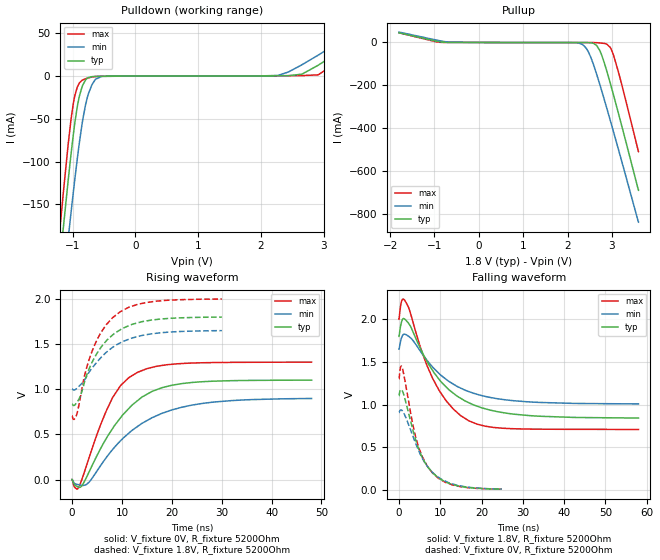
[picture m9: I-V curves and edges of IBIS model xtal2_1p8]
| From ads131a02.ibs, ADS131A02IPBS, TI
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|   xtal2_1p8 Model
[Model]   xtal2_1p8
Model_type   Output
Polarity   Inverting
Vmeas = 0.9
Vref = 0
Cref = 2pF
Rref = 5200
|   typ   min   max
|   (nom PVT)   (fast PVT)   (slow PVT)
C_comp   1.642e-12   1.633e-12   1.659e-12
| Where nom  PVT is Nominal Process, 1.8V, 27C
|   Fast PVT is Strong Process,  2V, -40C
|   Slow PVT is Weak Process,   1.65V, 125C
[Voltage Range]   1.8   1.65   2
|Junction Temperature
[Temperature Range]   27   125   -40
[Pullup Reference]   1.8   1.65   2
[Pulldown Reference]   0   0   0
[Power Clamp Reference]   1.8   1.65   2
[GND Clamp Reference]   0   0   0
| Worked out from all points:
|   slope of the pulldown table from 0 to 0.27 V, typ, clamps not added: 3.11 kohm
|   slope of the pullup table from 0 to 0.27 V, typ, clamps not added: 3.11 kohm
|   falling waveform, V_fixture 1.8V, R_fixture 5200Ohm: 20-80 % time 10.7ns typ, 11.1ns min, 8.07ns max; typ from 1.8 V to 0.842 V
|   rising waveform, V_fixture 0V, R_fixture 5200Ohm: 20-80 % time 8.7ns typ, 11.4ns min, 6.19ns max; typ from 0 V to 1.1 V
|   rising waveform, V_fixture 1.8V, R_fixture 5200Ohm: 20-80 % time 6.01ns typ, 7.06ns min, 5.43ns max; typ from 0.834 V to 1.79 V
|   falling waveform, V_fixture 0V, R_fixture 5200Ohm: 20-80 % time 5.28ns typ, 5.86ns min, 4.74ns max; typ from 1.1 V to 0.008 V
[Pulldown]
|   Voltage   I(typ)   I(min)   I(max)
-1.8V     -689.5mA   -725.3mA   -679.6mA
-1.216V   -227.2mA   -291.2mA   -188.7mA
-1.145V   -174.2mA   -240.9mA   -133.1mA
-1.073V   -122.5mA   -190.9mA   -80.24mA
-988mV    -67.27mA   -134.6mA   -31.2mA
-920mV    -33mA      -92.84mA   -11.74mA
-840mV    -10.65mA   -51.17mA   -4.594mA
-694.5mV  -724.7uA   -10.25mA   -1.163mA
-537.7mV  -196.1uA   -451.9uA   -234.3uA
2.272V    329.2uA    732.2uA    303.8uA
2.914V    12.62mA    24.45mA    1.392mA
3.6V      45.3mA     55.53mA    34.6mA
[Pullup]
|   Voltage   I(typ)   I(min)   I(max)
-1.8V     45.24mA    48.61mA    45.22mA
-853.2mV  2.132mA    7.04mA     429.8uA
2.224V    -250.1uA   -1.029mA   -357.3uA
2.324V    -269.6uA   -7.801mA   -357.9uA
2.475V    -699.5uA   -46.15mA   -368.8uA
2.662V    -15.95mA   -152mA     -1.072mA
2.772V    -60.12mA   -227.1mA   -3.044mA
2.888V    -135.7mA   -309.5mA   -8.122mA
2.984V    -206.2mA   -379.5mA   -31.46mA
3.034V    -243.7mA   -416mA     -57.5mA
3.171V    -350.1mA   -518mA     -156.8mA
3.6V      -691mA     -840.4mA   -510.4mA
[Ramp]
R_load = 5200
|   typ   min   max
dV/dt_r   0.660428/8.73874e-09   0.540772/1.15508e-08   0.779587/6.21968e-09
dV/dt_f   0.577509/1.08656e-08   0.387239/1.12171e-08   0.776401/8.09564e-09
[Falling Waveform]
V_fixture = 1.8V
V_fixture_min = 1.65V
V_fixture_max = 2V
R_fixture = 5200Ohm
|   Time   V(typ)   V(min)   V(max)
0s        1.8V       1.65V      2V
626.3ps   1.972V     1.785V     2.213V
1.396ns   2.002V     1.825V     2.222V
2.522ns   1.939V     1.793V     2.111V
5.623ns   1.613V     1.594V     1.609V
8.119ns   1.401V     1.441V     1.309V
11.36ns   1.209V     1.298V     1.048V
16.93ns   1.021V     1.152V     809.2mV
30.93ns   873.1mV    1.033V     712.8mV
58.02ns   841.7mV    1.007V     707.9mV
[Rising Waveform]
V_fixture = 0V
V_fixture_min = 0V
V_fixture_max = 0V
R_fixture = 5200Ohm
|   Time   V(typ)   V(min)   V(max)
0s        1.779uV    13.16uV    582nV
485.6ps   -60.15mV   -42.36mV   -84.12mV
1.314ns   -85.32mV   -57.05mV   -86.43mV
3.335ns   76.32mV    -32.93mV   230.6mV
8.119ns   564.1mV    331.6mV    906mV
9.712ns   683.1mV    428.1mV    1.039V
13.1ns    870.8mV    585.6mV    1.184V
18.02ns   1.015V     731.5mV    1.26V
26.02ns   1.081V     840mV      1.29V
48.02ns   1.098V     895.6mV    1.297V
[Rising Waveform]
V_fixture = 1.8V
V_fixture_min = 1.65V
V_fixture_max = 2V
R_fixture = 5200Ohm
|   Time   V(typ)   V(min)   V(max)
0s        833.9mV    1.002V     704.3mV
384.7ps   818mV      988.3mV    664.6mV
939.1ps   851.6mV    1.008V     721mV
1.699ns   929.6mV    1.048V     922mV
2.765ns   1.13V      1.125V     1.207V
4.564ns   1.355V     1.27V      1.494V
8.119ns   1.597V     1.46V      1.789V
11.36ns   1.7V       1.55V      1.903V
14.93ns   1.753V     1.601V     1.957V
30.02ns   1.795V     1.645V     1.994V
[Falling Waveform]
V_fixture = 0V
V_fixture_min = 0V
V_fixture_max = 0V
R_fixture = 5200Ohm
|   Time   V(typ)   V(min)   V(max)
0s        1.102V     904.1mV    1.301V
384.8ps   1.173V     936mV      1.439V
700.8ps   1.168V     931.8mV    1.443V
3.476ns   680.9mV    614.5mV    734.5mV
4.564ns   505.3mV    480.8mV    530.6mV
6.752ns   285.2mV    282.4mV    285.1mV
8.119ns   202.3mV    204.6mV    196.2mV
11.36ns   92.33mV    98.6mV     84.23mV
14.02ns   48.55mV    53.72mV    45.58mV
24.93ns   7.586mV    7.881mV    7.533mV
